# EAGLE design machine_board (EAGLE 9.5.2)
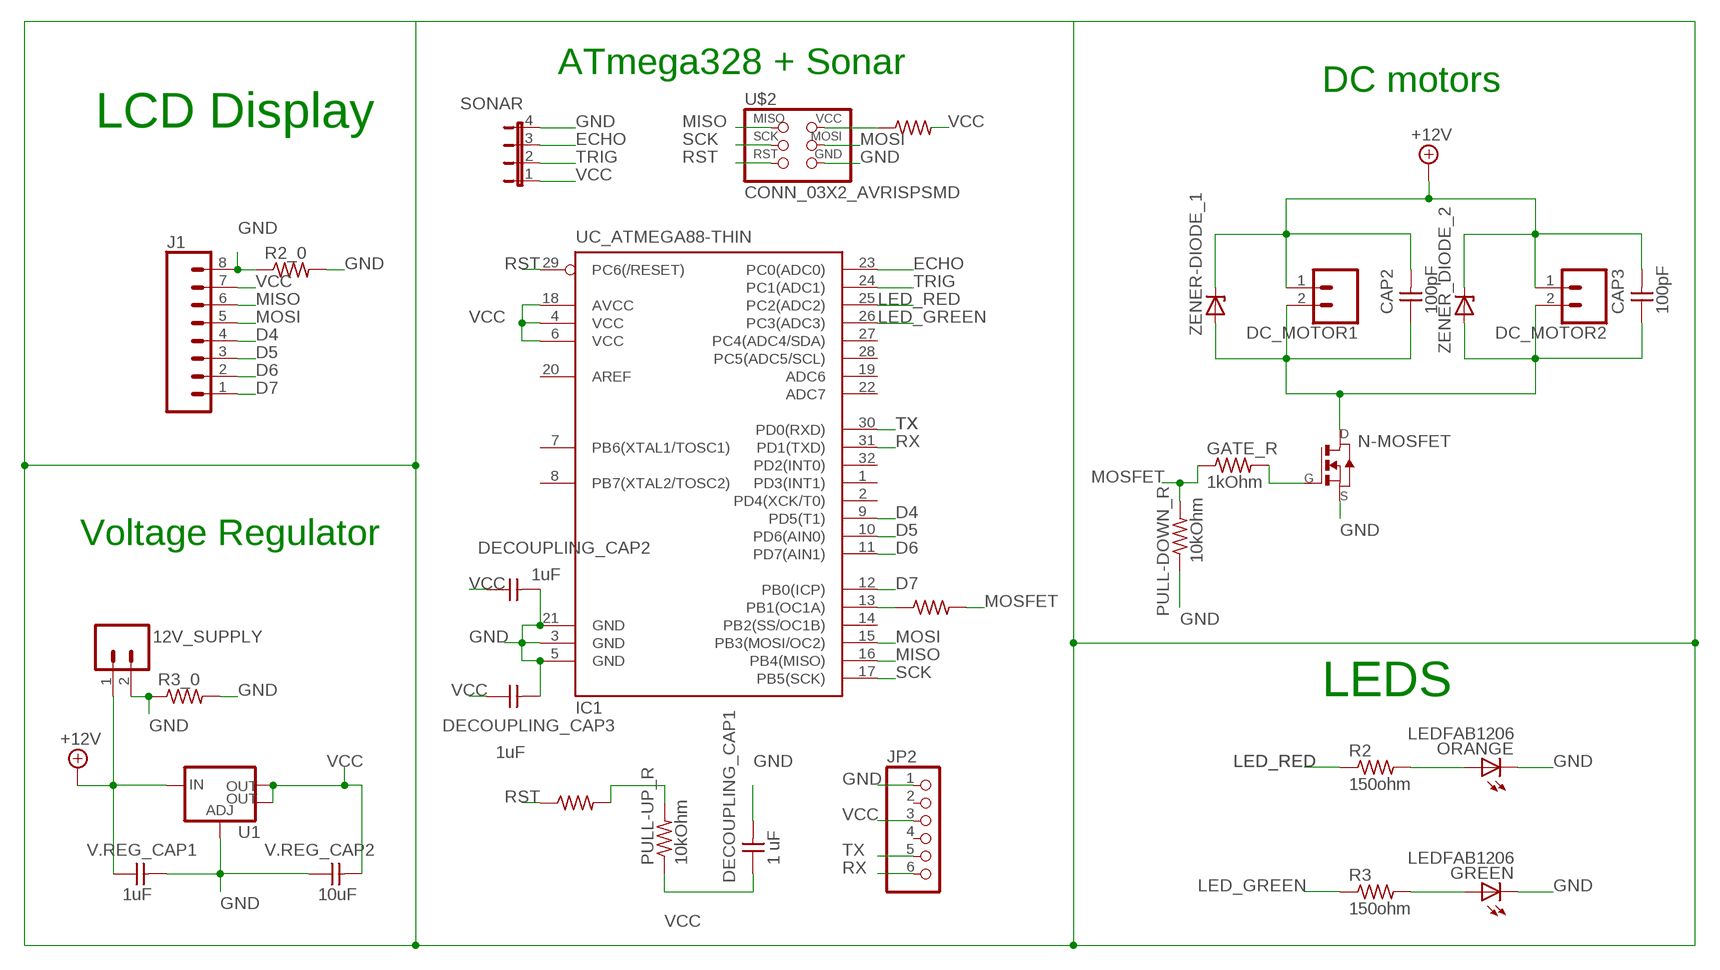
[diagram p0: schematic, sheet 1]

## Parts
0_RES  R1206FAB  [R1206FAB]
12V_SUPPLY  CONN_025MM  [SCREWTERMINAL-5MM-2]
CAP2  100pF  CAP_UNPOLARIZEDFAB  [C1206FAB]
CAP3  100pF  CAP_UNPOLARIZEDFAB  [C1206FAB]
DC_MOTOR1  CONN_025MM  [SCREWTERMINAL-5MM-2]
DC_MOTOR2  CONN_025MM  [SCREWTERMINAL-5MM-2]
DECOUPLING_CAP1  1 uF  CAP_UNPOLARIZEDFAB  [C1206FAB]
DECOUPLING_CAP2  1uF  CAP_UNPOLARIZEDFAB  [C1206FAB]
DECOUPLING_CAP3  1uF  CAP_UNPOLARIZEDFAB  [C1206FAB]
GATE_R  1kOhm  R1206FAB  [R1206FAB]
GREEN  LEDFAB1206  [LED1206FAB]
IC1  UC_ATMEGA88-THIN  [TQFP32-08THIN]
J1  CONN_08"  [1X08]
JP2  PINHD-1X6  [1X06]
N-MOSFET  MOSFET_NSOT23  [SOT-23]
ORANGE  LEDFAB1206  [LED1206FAB]
PULL-DOWN_R  10kOhm  R1206FAB  [R1206FAB]
PULL-UP_R  10kOhm  R1206FAB  [R1206FAB]
R1_0  R1206FAB  [R1206FAB]
R2  150ohm  R1206FAB  [R1206FAB]
R2_0  R1206FAB  [R1206FAB]
R3  150ohm  R1206FAB  [R1206FAB]
R3_0  R1206FAB  [R1206FAB]
R4_0  R1206FAB  [R1206FAB]
SONAR  JP4E  [JP4]
U1  VR_REGULATOR_LM1117SOT223  [SOT223]
U$2  CONN_03X2_AVRISPSMD  [2X03SMD]
V.REG_CAP1  1uF  CAP_UNPOLARIZEDFAB  [C1206FAB]
V.REG_CAP2  10uF  CAP_UNPOLARIZEDFAB  [C1206FAB]
ZENER-DIODE_1  DIODE_ZENERSOD123  [SOD123]
ZENER_DIODE_2  DIODE_ZENERSOD123  [SOD123]

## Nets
+12V: 12V_SUPPLY.1 CAP2.2 CAP3.2 DC_MOTOR1.1 DC_MOTOR2.1 U1.3(IN) V.REG_CAP1.1 ZENER-DIODE_1.CATHODE ZENER_DIODE_2.CATHODE
D4: IC1.9(PD5(T1)) J1.4
D5: IC1.10(PD6(AIN0)) J1.3
D6: IC1.11(PD7(AIN1)) J1.2
D7: IC1.12(PB0(ICP)) J1.1
ECHO: IC1.23(PC0(ADC0)) SONAR.3
GND: 12V_SUPPLY.2 DECOUPLING_CAP1.2 DECOUPLING_CAP2.2 DECOUPLING_CAP3.2 GREEN.2(C) IC1.3(GND) IC1.5(GND) IC1.21(GND) J1.8 JP2.1 N-MOSFET.2(S) ORANGE.2(C) PULL-DOWN_R.1 R2_0.1 R2_0.2 R3_0.1 R3_0.2 SONAR.4 U1.1(ADJ) U$2.6(GND) V.REG_CAP1.2 V.REG_CAP2.1
LED_GREEN: IC1.26(PC3(ADC3)) R3.1
LED_RED: IC1.25(PC2(ADC2)) R2.1
MISO: IC1.16(PB4(MISO)) J1.6 U$2.1(MISO)
MOSFET: 0_RES.2 GATE_R.1 PULL-DOWN_R.2
MOSI: IC1.15(PB3(MOSI/OC2)) J1.5 U$2.4(MOSI)
N$2: ORANGE.1(A) R2.2
N$3: GREEN.1(A) R3.2
N$4: 0_RES.1 IC1.13(PB1(OC1A))
N$5: CAP2.1 CAP3.1 DC_MOTOR1.2 DC_MOTOR2.2 N-MOSFET.1(D) ZENER-DIODE_1.ANODE ZENER_DIODE_2.ANODE
N$6: GATE_R.2 N-MOSFET.3(G)
N$8: R1_0.1 U$2.2(VCC)
RST: IC1.29(PC6(/RESET)) PULL-UP_R.2 R4_0.1 R4_0.2 U$2.5(RST)
RX: IC1.31(PD1(TXD)) JP2.6
SCK: IC1.17(PB5(SCK)) U$2.3(SCK)
TRIG: IC1.24(PC1(ADC1)) SONAR.2
TX: IC1.30(PD0(RXD)) JP2.5
VCC: DECOUPLING_CAP1.1 DECOUPLING_CAP2.1 DECOUPLING_CAP3.1 IC1.4(VCC) IC1.6(VCC) IC1.18(AVCC) J1.7 JP2.3 PULL-UP_R.1 R1_0.2 SONAR.1 U1.2(OUT) U1.4(OUT) V.REG_CAP2.2
Unconnected: IC1.1(PD3(INT1)) IC1.2(PD4(XCK/T0)) IC1.7(PB6(XTAL1/TOSC1)) IC1.8(PB7(XTAL2/TOSC2)) IC1.14(PB2(SS/OC1B)) IC1.19(ADC6) IC1.20(AREF) IC1.22(ADC7) IC1.27(PC4(ADC4/SDA)) IC1.28(PC5(ADC5/SCL)) IC1.32(PD2(INT0)) JP2.2 JP2.4

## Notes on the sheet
- ATmega328 + Sonar
- DC motors
- LCD Display
- Voltage Regulator
- LEDS

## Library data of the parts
0_RES GATE_R PULL-DOWN_R PULL-UP_R R1_0 R2 R2_0 R3 R3_0 R4_0 = fab:R: Resistor (US Symbol)
12V_SUPPLY DC_MOTOR1 DC_MOTOR2 = SparkFun-Connectors:CONN_02: Multi connection point. Often used as Generic Header-pin footprint for 0.1 inch spaced/style header connections; SF_SKU: PRT-08432
CAP2 CAP3 DECOUPLING_CAP1-DECOUPLING_CAP3 V.REG_CAP1 V.REG_CAP2 = fab:CAP_UNPOLARIZED
GREEN ORANGE = fab:LED: LED
IC1 = fab:UC_ATMEGA88-THIN
J1 = SparkFun-Connectors:CONN_08: Multi connection point. Often used as Generic Header-pin footprint for 0.1 inch spaced/style header connections On any of the 0.1 inch spaced packages, you can populate with these: Break Away Headers - Straight (PRT-00116) Break Away Male Headers - Right Angle (PRT-00553) Female Headers (PRT-00115)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; PROD_ID: CONN-08438
JP2 = pinhead:PINHD-1X6: PIN HEADER
N-MOSFET = fab:MOSFET_N: MOS FET
SONAR = jumper:JP4E: JUMPER
U1 = fab:VR_REGULATOR_LM1117: Voltage Regulator LM1117 Standard adjustable voltage regulator but in SMD form. Spark Fun Electronics SKU : COM-00595; PROD_ID: VREG-08170
U$2 = fab:CONN_03X2_AVRISP
ZENER-DIODE_1 ZENER_DIODE_2 = fab:DIODE_ZENER: zener diode

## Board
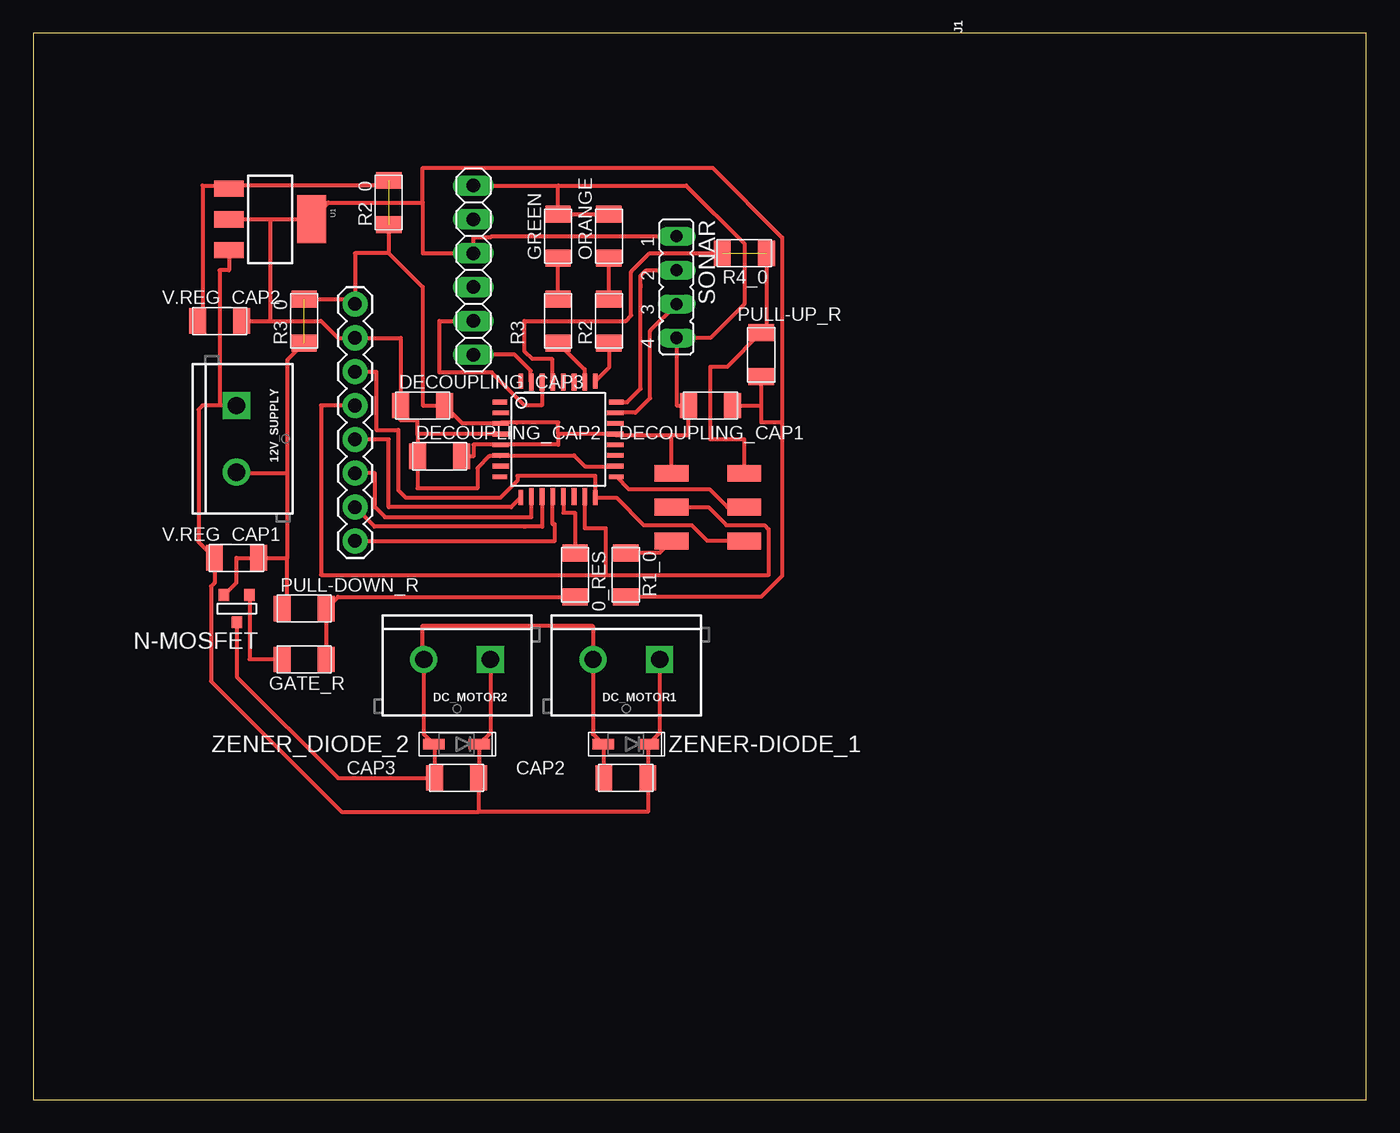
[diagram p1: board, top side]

Size 100 x 80 mm. Coordinates in mm from the lower left corner, seen from the top.
Outline: 0,0 100,0 100,80 0,80 0,0
Copper layers (1*16): Top 0.035mm / dielectric 1.5mm / Bottom 0.035mm
Design rules "default *": minimum track width 12mil, minimum drill 32mil, track to track 16mil, track to pad 16mil, pad to pad 16mil, via to via 16mil, smd to smd 16mil, copper to edge 16mil, drill to drill 16mil, minimum pad ring 10mil, minimum via ring 8mil, stop-mask expansion 4mil, vias tented up to drill 0mil, thermal gap 10mil

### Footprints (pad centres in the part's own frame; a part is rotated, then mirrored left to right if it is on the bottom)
R1206FAB = smd 1.27 x 1.905: 1 -1.651,0; 2 1.651,0
SCREWTERMINAL-5MM-2 = drill 1.3 pad 2.032 square: 1 0,0 | drill 1.3 pad 2.032: 2 5,0
C1206FAB = smd 1.27 x 1.905: 1 -1.651,0; 2 1.651,0
LED1206FAB = smd 1.27 x 1.905: 1 -1.651,0; 2 1.651,0
TQFP32-08THIN = smd 1.118 x 0.356: 1 -4.369,2.8; 8 -4.369,-2.8; 17 4.369,-2.8; 24 4.369,2.8 | smd 1.27 x 0.356: 2 -4.293,2; 3 -4.293,1.2; 4 -4.293,0.4; 5 -4.293,-0.4; 6 -4.293,-1.2; 7 -4.293,-2; 18 4.293,-2; 19 4.293,-1.2; 20 4.293,-0.4; 21 4.293,0.4; 22 4.293,1.2; 23 4.293,2 | smd 0.356 x 1.118: 9 -2.8,-4.369; 16 2.8,-4.369; 25 2.8,4.369; 32 -2.8,4.369 | smd 0.356 x 1.27: 10 -2,-4.293; 14 1.2,-4.293; 15 2,-4.293; 26 2,4.293; 27 1.2,4.293; 31 -2,4.293 | smd 0.35 x 1.27: 11 -1.2,-4.293; 12 -0.4,-4.293; 13 0.4,-4.293; 28 0.4,4.293; 29 -0.4,4.293; 30 -1.2,4.293
1X08 = drill 1.016 pad 1.88: 1 0,0; 2 2.54,0; 3 5.08,0; 4 7.62,0; 5 10.16,0; 6 12.7,0; 7 15.24,0; 8 17.78,0
1X06 = drill 1.016 long: 1 -6.35,0; 2 -3.81,0; 3 -1.27,0; 4 1.27,0; 5 3.81,0; 6 6.35,0
SOT-23 = smd 0.787 x 0.889: 1 0.025,-1.016; 2 -0.94,1.016; 3 0.991,1.016
JP4 = drill 0.914 long: 1 -3.81,0; 2 -1.27,0; 3 1.27,0; 4 3.81,0
SOT223 = smd 1.219 x 2.235: 1 -2.311,-3.099; 2 0,-3.099; 3 2.311,-3.099 | smd 3.6 x 2.2: 4 0,3.099
2X03SMD = smd 2.54 x 1.27: 1 -2.54,2.54; 2 2.92,2.54; 3 -2.54,0; 4 2.92,0; 5 -2.54,-2.54; 6 2.92,-2.54
SOD123 = smd 1.6 x 0.8: ANODE 1.7,0; CATHODE -1.7,0

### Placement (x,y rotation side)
0_RES  40.64,39.37 270 top
12V_SUPPLY  15.24,52.07 270 top
CAP2  44.45,24.13 0 top
CAP3  31.75,24.13 0 top
DC_MOTOR1  46.99,33.02 180 top
DC_MOTOR2  34.29,33.02 180 top
DECOUPLING_CAP1  50.8,52.07 180 top
DECOUPLING_CAP2  30.48,48.26 0 top
DECOUPLING_CAP3  29.21,52.07 0 top
GATE_R  20.32,33.02 180 top
GREEN  39.37,64.77 90 top
IC1  39.37,49.53 0 top
J1  24.13,41.91 90 top
JP2  33.02,62.23 270 top
N-MOSFET  15.24,36.83 0 top
ORANGE  43.18,64.77 90 top
PULL-DOWN_R  20.32,36.83 0 top
PULL-UP_R  54.61,55.88 90 top
R1_0  44.45,39.37 270 top
R2  43.18,58.42 90 top
R2_0  26.67,67.31 90 top
R3  39.37,58.42 90 top
R3_0  20.32,58.42 90 top
R4_0  53.34,63.5 180 top
SONAR  48.26,60.96 270 top
U1  17.78,66.04 270 top
U$2  50.8,44.45 180 top
V.REG_CAP1  15.24,40.64 0 top
V.REG_CAP2  13.97,58.42 0 top
ZENER-DIODE_1  44.45,26.67 180 top
ZENER_DIODE_2  31.75,26.67 180 top

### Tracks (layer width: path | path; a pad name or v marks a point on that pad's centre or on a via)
+12V
  Top 0.305: 12V_SUPPLY.1 13.97,52.07 | 13.97,52.07 12.7,52.07 12.39,51.77 12.39,41.83 V.REG_CAP1.1 13.59,38.76 13.34,38.51 13.34,31.38 23.12,21.59 33.4,21.59 | U1.3 14.68,62.23 13.97,62.23 13.97,52.07 | DC_MOTOR2.1 34.29,27.51 ZENER_DIODE_2.CATHODE 33.45,24.18 CAP3.2 33.4,21.59 | DC_MOTOR1.1 46.99,27.51 ZENER-DIODE_1.CATHODE 46.1,26.62 CAP2.2 46.1,21.59 33.4,21.59
D4
  Top 0.305: IC1.9 35.86,44.45 26.67,44.45 26.67,49.53 J1.4
D5
  Top 0.305: J1.3 25.63,46.99 25.63,44.45 26.39,43.69 37.37,43.69 IC1.10
D6
  Top 0.305: J1.2 25.6,42.98 36.83,42.98 36.92,42.98 38.17,42.98 38.17,44.23 38.17,44.45 IC1.11
D7
  Top 0.305: IC1.12 38.97,43.18 39.13,43.18 39.13,41.91 J1.1
ECHO
  Top 0.305: SONAR.3 48.26,59.66 46.28,57.68 46.28,52.63 45.18,51.53 IC1.23
GND  (2 unrouted)
  Top 0.305: 47.42,47.45 U$2.6 47.88,49.87 | 43.56,66.42 ORANGE.2 GREEN.2 39.37,68.58 | 47.88,49.87 43.66,49.87 IC1.21 39.37,49.93 | N-MOSFET.2 14.05,38.1 | 19.05,40.64 V.REG_CAP1.2 15.24,40.64 15.24,38.79 N-MOSFET.2 | 14.3,38.1 N-MOSFET.2 | 39.37,68.58 48.99,68.58 53.34,64.23 53.34,59.69 50.8,57.15 SONAR.4 48.26,52.07 DECOUPLING_CAP1.2 49.15,49.87 47.88,49.87 | 26.67,63.5 29.21,60.96 29.21,52.07 DECOUPLING_CAP3.2 32.2,50.73 IC1.3 35.08,50.79 36.27,50.79 36.27,50.8 39.37,50.8 39.37,49.93 | JP2.1 39.37,68.58 | V.REG_CAP2.1 12.7,58.8 12.7,68.58 14.45,68.58 U1.1 14.91,68.58 26.29,68.58 R2_0.2 | R2_0.1 26.67,63.5 | R3_0.1 19.05,55.5 19.05,46.99 | 12V_SUPPLY.2 15.32,46.99 19.05,46.99 | 39.37,49.93 39.37,49.13 IC1.5 33.02,49.13 33.02,48.26 DECOUPLING_CAP2.2 | R3_0.2 24.13,60.07 J1.8 24.13,63.5 26.67,63.5 | 19.05,46.99 19.05,40.64 | PULL-DOWN_R.1 19.05,37.21 19.05,40.64
LED_GREEN
  Top 0.305: R3.1 41.37,54.77 IC1.26
LED_RED
  Top 0.305: R2.1 43.18,54.91 IC1.25
MISO
  Top 0.305: U$2.1 50.58,41.91 49.38,43.1 45.8,43.1 43.74,45.16 IC1.16 42.17,46.79 36.31,46.79 36.31,46.43 35.04,45.16 27.94,45.16 27.38,45.72 27.38,50.24 25.73,50.24 25.73,54.61 J1.6
MOSFET
  Top 0.305: GATE_R.1 PULL-DOWN_R.2 22.86,37.72 0_RES.2
MOSI
  Top 0.305: U$2.4 50.65,44.45 51.99,43.1 54.84,43.1 55.17,42.78 55.17,39.37 42.94,39.37 | J1.5 21.59,52.07 21.59,39.37 42.94,39.37 | 42.94,39.37 42.94,42.87 41.37,42.87 IC1.15
N$2
  Top 0.305: R2.2 ORANGE.1
N$3
  Top 0.305: R3.2 GREEN.1
N$4
  Top 0.305: IC1.13 39.77,44.04 40.64,44.04 0_RES.1
N$5
  Top 0.305: N-MOSFET.1 15.27,31.73 22.86,24.13 CAP3.1 30.1,26.62 ZENER_DIODE_2.ANODE 29.29,27.43 DC_MOTOR2.2 29.21,33.1 29.21,35.56 41.91,35.56 41.99,35.48 DC_MOTOR1.2 41.99,27.43 ZENER-DIODE_1.ANODE 42.8,26.62 CAP2.1
N$6
  Top 0.305: GATE_R.2 16.23,33.02 N-MOSFET.3
N$8
  Top 0.305: U$2.2 46.99,41.02 R1_0.1
RST  (1 unrouted)
  Top 0.305: IC1.29 38.9,53.89 38.9,55.58 37.43,55.58 36.83,56.17 36.83,58.42 44.45,58.42 44.86,58.83 44.86,62.11 46.25,63.5 R4_0.2 | R4_0.1 54.99,57.91 PULL-UP_R.2 52.07,54.99 50.8,54.99 50.8,49.53 53.34,49.53 U$2.5
RX
  Top 0.305: IC1.31 37.31,53.89 37.31,54.69 36.12,55.88 JP2.6
SCK
  Top 0.305: U$2.3 52.07,44.45 50.72,45.8 44.67,45.8 IC1.17
TRIG
  Top 0.305: IC1.24 44.56,52.33 45.57,53.34 45.57,60.96 45.57,61.11 45.57,61.81 45.98,62.23 SONAR.2
TX
  Top 0.305: JP2.5 30.48,58.42 30.48,54.56 34.38,54.56 36.87,52.07 38.1,52.07 38.17,52.14 IC1.30
VCC
  Top 0.305: R1_0.2 54.61,37.72 56.19,39.29 56.19,50.8 | 56.19,50.8 56.19,64.68 50.97,69.9 29.21,69.9 29.21,67.31 | 56.19,50.8 54.61,50.8 54.61,52.07 | U1.2 17.78,66.04 | 17.78,66.04 U1.4 22.15,67.31 29.21,67.31 | V.REG_CAP2.2 17.78,58.42 | 17.78,66.04 17.78,58.42 | 17.78,58.42 21.59,58.42 22.86,57.15 J1.7 27.56,57.15 DECOUPLING_CAP3.1 27.56,50.95 28.83,50.95 28.83,49.93 | IC1.4 28.83,49.93 | 28.83,49.93 DECOUPLING_CAP2.1 28.83,45.87 33.33,45.87 33.33,47.38 34.21,48.27 35.01,48.27 IC1.6 40.57,48.33 41.4,47.51 43.64,47.51 IC1.18 | 29.21,67.31 29.21,63.5 JP2.3 33.02,64.72 34.33,64.72 34.38,64.77 SONAR.1 | PULL-UP_R.1 54.61,52.07 | DECOUPLING_CAP1.1 54.61,52.07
